(* Logix 5000 Program export KEP; software revision 30.00; part 14 of 15 *)
(* tags used below, declared in another part *)
   B256_CtoE : B256_CtoE;
   B256_CtoS : B256_CtoS;
   B256_DINTtoE : B256_DINTtoE;
   B256_EtoC : B256_EtoC;
   B256_EtoDINT : B256_EtoDINT;
   B256_EtoL : B256_EtoL;
   B256_StoC : B256_StoC;
   B256_StoC_LE : B256_StoC_LE;
   EdDSA_INTERNAL : EdDSA_INTERNAL[5];
   EdDSA_STATES : EdDSA_STATECTRL[15];
   InternalFlags : InternalFlags[5];
   InternalFlag_CreateNewKsPrime : BOOL;
   InternalFlag_KsEqualKsPrimeStatus : BOOL;
   InternalFlag_KsExists : BOOL;
   MyNodeNumber : DINT;
   POINT_DEC : POINT_DEC;
   POINT_ENC : POINT_ENC;
   POINT_MUL : POINT_MUL;
   PRN : STRING;
   PRNG : PRNG;
   PRNG_Constant : STRING;
   PRNG_Counter : LINT;
   PRNG_Seed : LINT[13];
   SHA512_SEQ : SHA512_SEQ;
   SignedMsgDest : INT;   // 0=None 1=Server 2=Client 3=All
   Temp_Processor_C1 : DINT[22];
   Temp_Processor_C10 : DINT[22];
   Temp_Processor_C11 : DINT[22];
   Temp_Processor_C12 : DINT[22];
   Temp_Processor_C2 : DINT[22];
   Temp_Processor_C3 : DINT[22];
   Temp_Processor_C4 : DINT[22];
   Temp_Processor_C5 : DINT[22];
   Temp_Processor_C6 : DINT[22];
   Temp_Processor_C7 : DINT[22];
   Temp_Processor_C8 : DINT[22];
   Temp_Processor_C9 : DINT[22];
   Temp_Processor_D1 : DINT[43];
   Temp_Processor_DINT1 : DINT[8];
   Temp_Processor_DINT2 : DINT[8];
   Temp_Processor_E1 : DINT[32];
   Temp_Processor_E2 : DINT[32];
   Temp_Processor_HASH : LINT[8];
   Temp_Processor_L : LINT[4];
   Temp_Processor_MSG : LINT[1600];
   Temp_Processor_P1 : POINT;
   Temp_Processor_P2 : POINT;
   Temp_Processor_P3 : POINT;
   Temp_Processor_P4 : POINT;
   T_INT1 : INT;
   WorkingNode : DINT;
   EdDSA_KS : DINT[8];
   EdDSA_KS_Prime : DINT[8];
   InternalFlag_KsID : LINT;
   InternalFlag_KsPrimeID : LINT;
   Wrk_InpA : DINT[2];
(* KEP, continued *)

ROUTINE PROCESSOR_STATE6   (* ladder *)
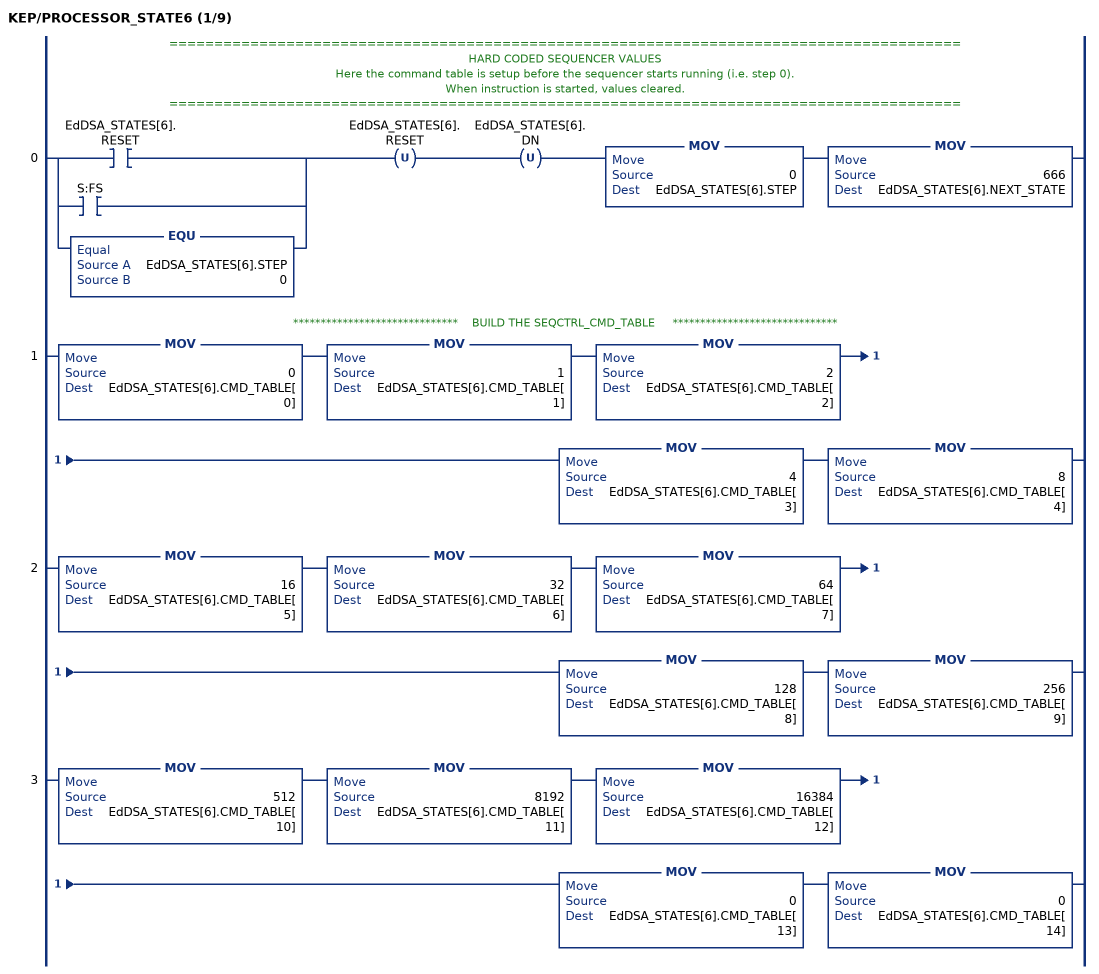
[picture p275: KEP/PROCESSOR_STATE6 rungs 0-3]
   // ========================================================================================
   // HARD CODED SEQUENCER VALUES
   // Here the command table is setup before the sequencer starts running (i.e. step 0).
   // When instruction is started, values cleared.
   // ========================================================================================
   0: [[XIC(EdDSA_STATES[6].RESET) ,XIC(S:FS) ] ,EQU(EdDSA_STATES[6].STEP,0) ]OTU(EdDSA_STATES[6].RESET)OTU(EdDSA_STATES[6].DN)MOV(0,EdDSA_STATES[6].STEP)MOV(666,EdDSA_STATES[6].NEXT_STATE);
   // ******************************    BUILD THE SEQCTRL_CMD_TABLE     ******************************
   1: MOV(0,EdDSA_STATES[6].CMD_TABLE[0])MOV(1,EdDSA_STATES[6].CMD_TABLE[1])MOV(2,EdDSA_STATES[6].CMD_TABLE[2])MOV(4,EdDSA_STATES[6].CMD_TABLE[3])MOV(8,EdDSA_STATES[6].CMD_TABLE[4]);
   2: MOV(16,EdDSA_STATES[6].CMD_TABLE[5])MOV(32,EdDSA_STATES[6].CMD_TABLE[6])MOV(64,EdDSA_STATES[6].CMD_TABLE[7])MOV(128,EdDSA_STATES[6].CMD_TABLE[8])MOV(256,EdDSA_STATES[6].CMD_TABLE[9]);
   3: MOV(512,EdDSA_STATES[6].CMD_TABLE[10])MOV(8192,EdDSA_STATES[6].CMD_TABLE[11])MOV(16384,EdDSA_STATES[6].CMD_TABLE[12])MOV(0,EdDSA_STATES[6].CMD_TABLE[13])MOV(0,EdDSA_STATES[6].CMD_TABLE[14]);
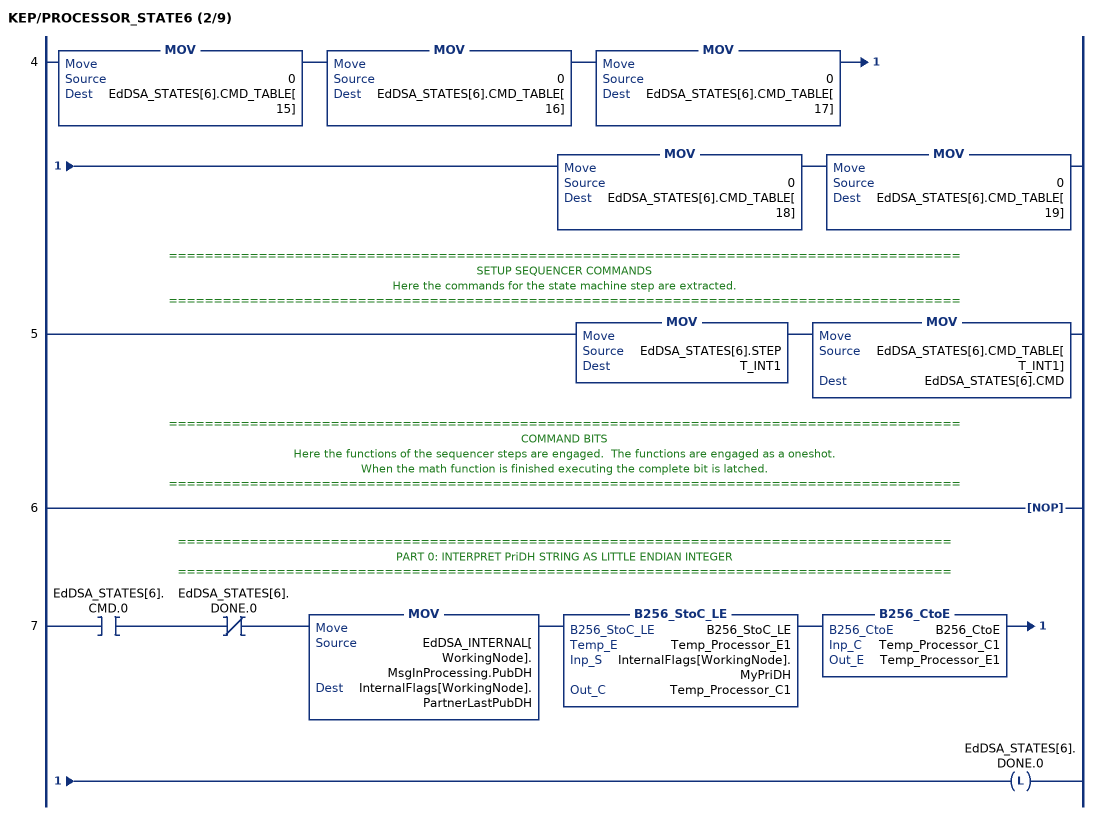
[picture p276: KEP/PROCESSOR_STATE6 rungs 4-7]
   4: MOV(0,EdDSA_STATES[6].CMD_TABLE[15])MOV(0,EdDSA_STATES[6].CMD_TABLE[16])MOV(0,EdDSA_STATES[6].CMD_TABLE[17])MOV(0,EdDSA_STATES[6].CMD_TABLE[18])MOV(0,EdDSA_STATES[6].CMD_TABLE[19]);
   // ========================================================================================
   // SETUP SEQUENCER COMMANDS
   // Here the commands for the state machine step are extracted.
   // ========================================================================================
   5: MOV(EdDSA_STATES[6].STEP,T_INT1)MOV(EdDSA_STATES[6].CMD_TABLE[T_INT1],EdDSA_STATES[6].CMD);
   // ========================================================================================
   // COMMAND BITS
   // Here the functions of the sequencer steps are engaged.  The functions are engaged as a oneshot.
   // When the math function is finished executing the complete bit is latched.
   // ========================================================================================
   6: NOP();
   // ======================================================================================
   // PART 0: INTERPRET PriDH STRING AS LITTLE ENDIAN INTEGER
   // ======================================================================================
   7: XIC(EdDSA_STATES[6].CMD.0)XIO(EdDSA_STATES[6].DONE.0)MOV(EdDSA_INTERNAL[WorkingNode].MsgInProcessing.PubDH,InternalFlags[WorkingNode].PartnerLastPubDH)B256_StoC_LE(B256_StoC_LE,Temp_Processor_E1,InternalFlags[WorkingNode].MyPriDH,Temp_Processor_C1)B256_CtoE(B256_CtoE,Temp_Processor_C1,Temp_Processor_E1)OTL(EdDSA_STATES[6].DONE.0);
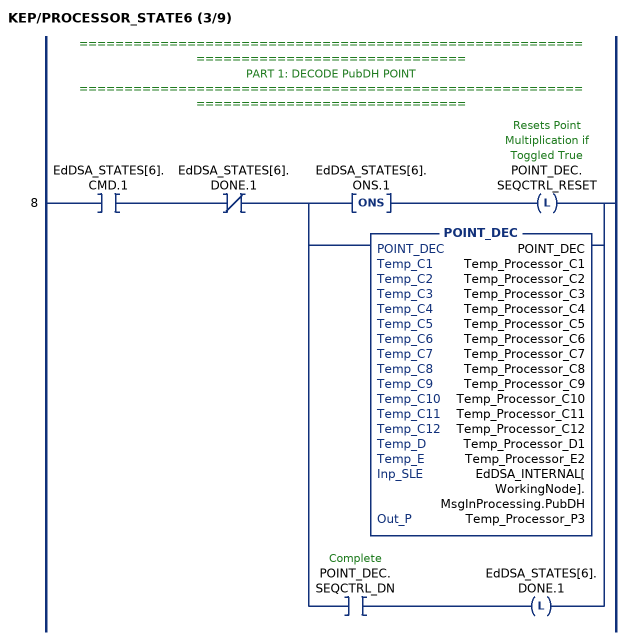
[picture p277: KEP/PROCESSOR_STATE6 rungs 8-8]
   // ======================================================================================
   // PART 1: DECODE PubDH POINT
   // ======================================================================================
   8: XIC(EdDSA_STATES[6].CMD.1)XIO(EdDSA_STATES[6].DONE.1)[ONS(EdDSA_STATES[6].ONS.1) OTL(POINT_DEC.SEQCTRL_RESET) ,POINT_DEC(POINT_DEC,Temp_Processor_C1,Temp_Processor_C2,Temp_Processor_C3,Temp_Processor_C4,Temp_Processor_C5,Temp_Processor_C6,Temp_Processor_C7,Temp_Processor_C8,Temp_Processor_C9,Temp_Processor_C10,Temp_Processor_C11,Temp_Processor_C12,Temp_Processor_D1,Temp_Processor_E2,EdDSA_INTERNAL[WorkingNode].MsgInProcessing.PubDH,Temp_Processor_P3) ,XIC(POINT_DEC.SEQCTRL_DN) OTL(EdDSA_STATES[6].DONE.1) ];
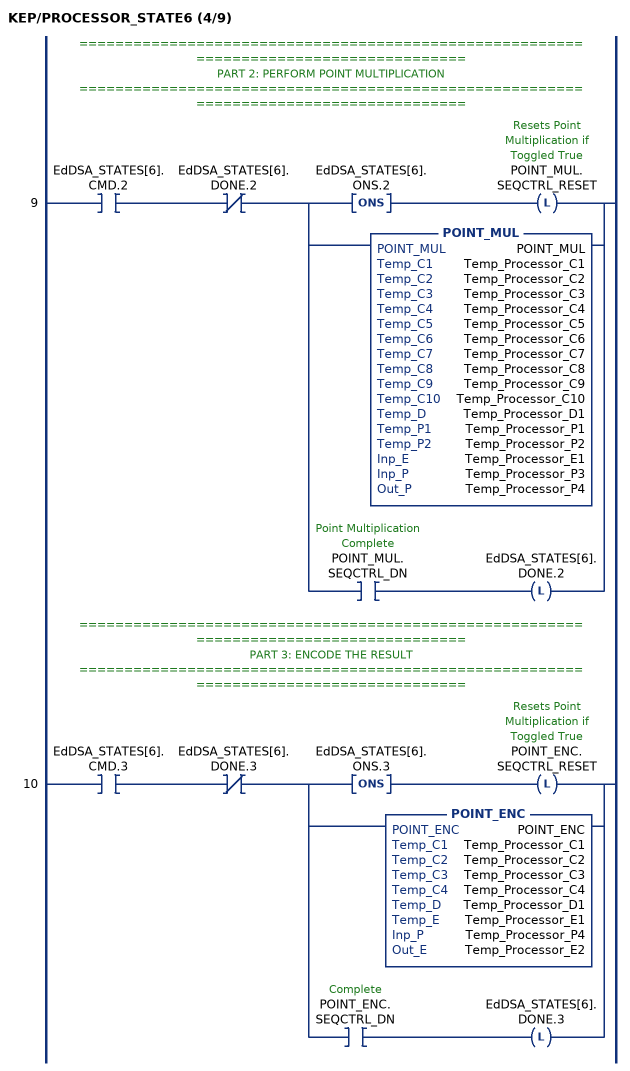
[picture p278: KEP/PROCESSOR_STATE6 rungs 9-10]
   // ======================================================================================
   // PART 2: PERFORM POINT MULTIPLICATION
   // ======================================================================================
   9: XIC(EdDSA_STATES[6].CMD.2)XIO(EdDSA_STATES[6].DONE.2)[ONS(EdDSA_STATES[6].ONS.2) OTL(POINT_MUL.SEQCTRL_RESET) ,POINT_MUL(POINT_MUL,Temp_Processor_C1,Temp_Processor_C2,Temp_Processor_C3,Temp_Processor_C4,Temp_Processor_C5,Temp_Processor_C6,Temp_Processor_C7,Temp_Processor_C8,Temp_Processor_C9,Temp_Processor_C10,Temp_Processor_D1,Temp_Processor_P1,Temp_Processor_P2,Temp_Processor_E1,Temp_Processor_P3,Temp_Processor_P4) ,XIC(POINT_MUL.SEQCTRL_DN) OTL(EdDSA_STATES[6].DONE.2) ];
   // ======================================================================================
   // PART 3: ENCODE THE RESULT
   // ======================================================================================
   10: XIC(EdDSA_STATES[6].CMD.3)XIO(EdDSA_STATES[6].DONE.3)[ONS(EdDSA_STATES[6].ONS.3) OTL(POINT_ENC.SEQCTRL_RESET) ,POINT_ENC(POINT_ENC,Temp_Processor_C1,Temp_Processor_C2,Temp_Processor_C3,Temp_Processor_C4,Temp_Processor_D1,Temp_Processor_E1,Temp_Processor_P4,Temp_Processor_E2) ,XIC(POINT_ENC.SEQCTRL_DN) OTL(EdDSA_STATES[6].DONE.3) ];
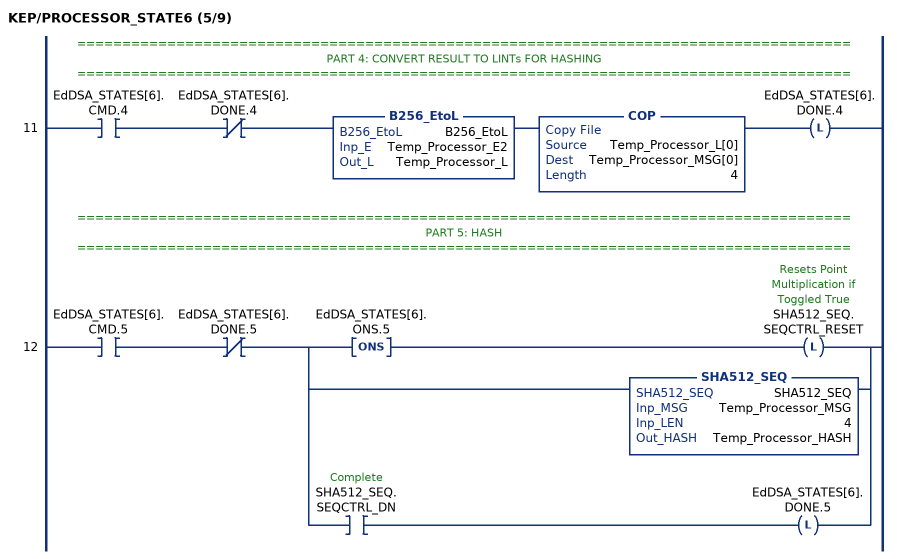
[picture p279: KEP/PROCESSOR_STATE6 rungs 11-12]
   // ======================================================================================
   // PART 4: CONVERT RESULT TO LINTs FOR HASHING
   // ======================================================================================
   11: XIC(EdDSA_STATES[6].CMD.4)XIO(EdDSA_STATES[6].DONE.4)B256_EtoL(B256_EtoL,Temp_Processor_E2,Temp_Processor_L)COP(Temp_Processor_L[0],Temp_Processor_MSG[0],4)OTL(EdDSA_STATES[6].DONE.4);
   // ======================================================================================
   // PART 5: HASH
   // ======================================================================================
   12: XIC(EdDSA_STATES[6].CMD.5)XIO(EdDSA_STATES[6].DONE.5)[ONS(EdDSA_STATES[6].ONS.5) OTL(SHA512_SEQ.SEQCTRL_RESET) ,SHA512_SEQ(SHA512_SEQ,Temp_Processor_MSG,4,Temp_Processor_HASH) ,XIC(SHA512_SEQ.SEQCTRL_DN) OTL(EdDSA_STATES[6].DONE.5) ];
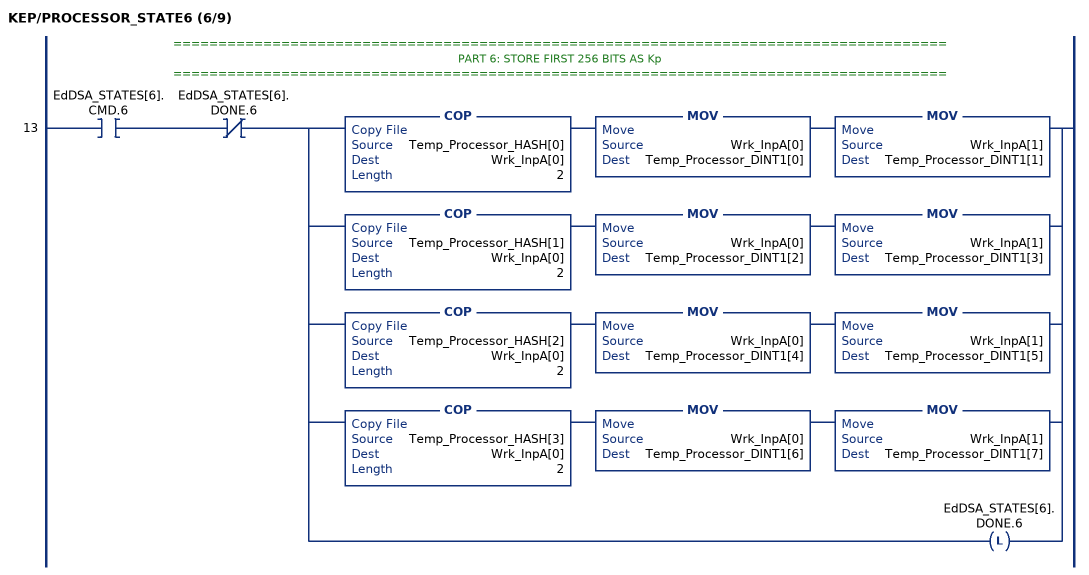
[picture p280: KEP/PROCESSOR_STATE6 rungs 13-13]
   // ======================================================================================
   // PART 6: STORE FIRST 256 BITS AS Kp
   // ======================================================================================
   13: XIC(EdDSA_STATES[6].CMD.6)XIO(EdDSA_STATES[6].DONE.6)[COP(Temp_Processor_HASH[0],Wrk_InpA[0],2) MOV(Wrk_InpA[0],Temp_Processor_DINT1[0]) MOV(Wrk_InpA[1],Temp_Processor_DINT1[1]) ,COP(Temp_Processor_HASH[1],Wrk_InpA[0],2) MOV(Wrk_InpA[0],Temp_Processor_DINT1[2]) MOV(Wrk_InpA[1],Temp_Processor_DINT1[3]) ,COP(Temp_Processor_HASH[2],Wrk_InpA[0],2) MOV(Wrk_InpA[0],Temp_Processor_DINT1[4]) MOV(Wrk_InpA[1],Temp_Processor_DINT1[5]) ,COP(Temp_Processor_HASH[3],Wrk_InpA[0],2) MOV(Wrk_InpA[0],Temp_Processor_DINT1[6]) MOV(Wrk_InpA[1],Temp_Processor_DINT1[7]) ,OTL(EdDSA_STATES[6].DONE.6) ];
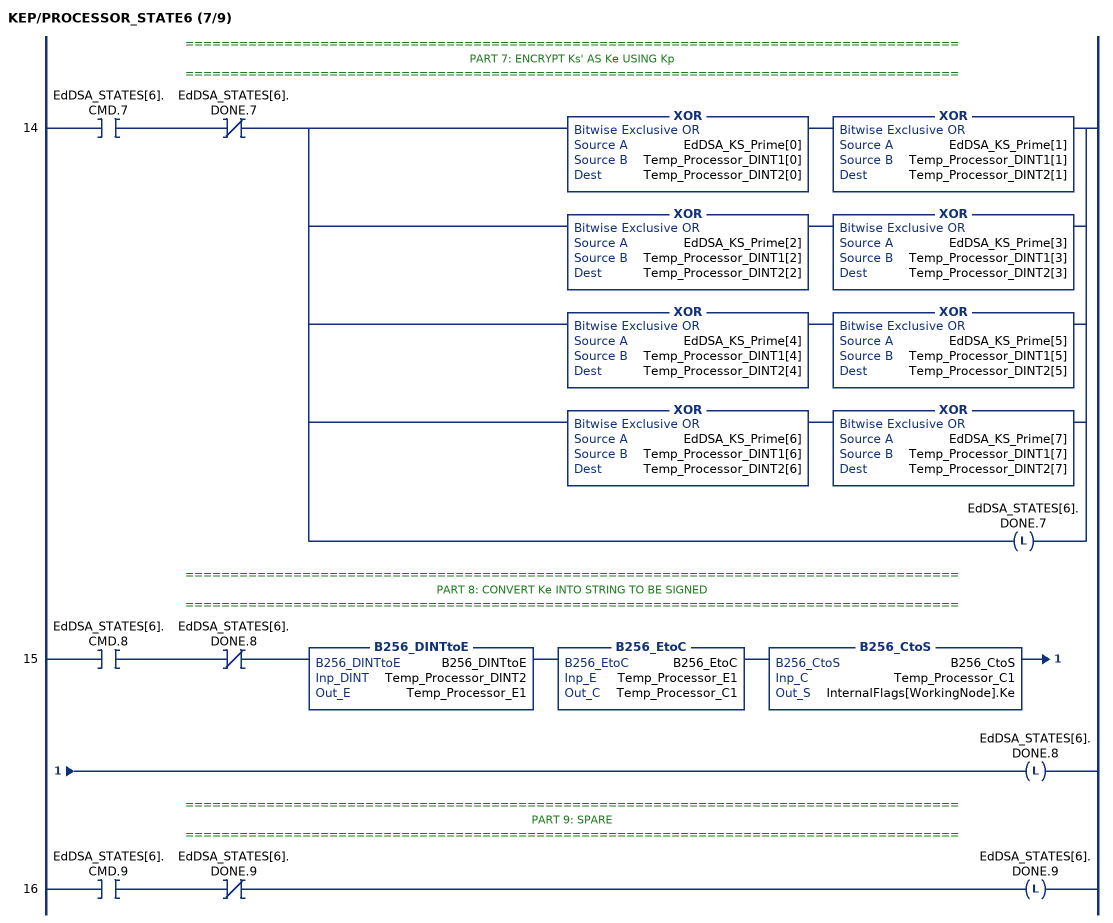
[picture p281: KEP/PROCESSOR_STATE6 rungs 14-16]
   // ======================================================================================
   // PART 7: ENCRYPT Ks' AS Ke USING Kp
   // ======================================================================================
   14: XIC(EdDSA_STATES[6].CMD.7)XIO(EdDSA_STATES[6].DONE.7)[XOR(EdDSA_KS_Prime[0],Temp_Processor_DINT1[0],Temp_Processor_DINT2[0]) XOR(EdDSA_KS_Prime[1],Temp_Processor_DINT1[1],Temp_Processor_DINT2[1]) ,XOR(EdDSA_KS_Prime[2],Temp_Processor_DINT1[2],Temp_Processor_DINT2[2]) XOR(EdDSA_KS_Prime[3],Temp_Processor_DINT1[3],Temp_Processor_DINT2[3]) ,XOR(EdDSA_KS_Prime[4],Temp_Processor_DINT1[4],Temp_Processor_DINT2[4]) XOR(EdDSA_KS_Prime[5],Temp_Processor_DINT1[5],Temp_Processor_DINT2[5]) ,XOR(EdDSA_KS_Prime[6],Temp_Processor_DINT1[6],Temp_Processor_DINT2[6]) XOR(EdDSA_KS_Prime[7],Temp_Processor_DINT1[7],Temp_Processor_DINT2[7]) ,OTL(EdDSA_STATES[6].DONE.7) ];
   // ======================================================================================
   // PART 8: CONVERT Ke INTO STRING TO BE SIGNED
   // ======================================================================================
   15: XIC(EdDSA_STATES[6].CMD.8)XIO(EdDSA_STATES[6].DONE.8)B256_DINTtoE(B256_DINTtoE,Temp_Processor_DINT2,Temp_Processor_E1)B256_EtoC(B256_EtoC,Temp_Processor_E1,Temp_Processor_C1)B256_CtoS(B256_CtoS,Temp_Processor_C1,InternalFlags[WorkingNode].Ke)OTL(EdDSA_STATES[6].DONE.8);
   // ======================================================================================
   // PART 9: SPARE
   // ======================================================================================
   16: XIC(EdDSA_STATES[6].CMD.9)XIO(EdDSA_STATES[6].DONE.9)OTL(EdDSA_STATES[6].DONE.9);
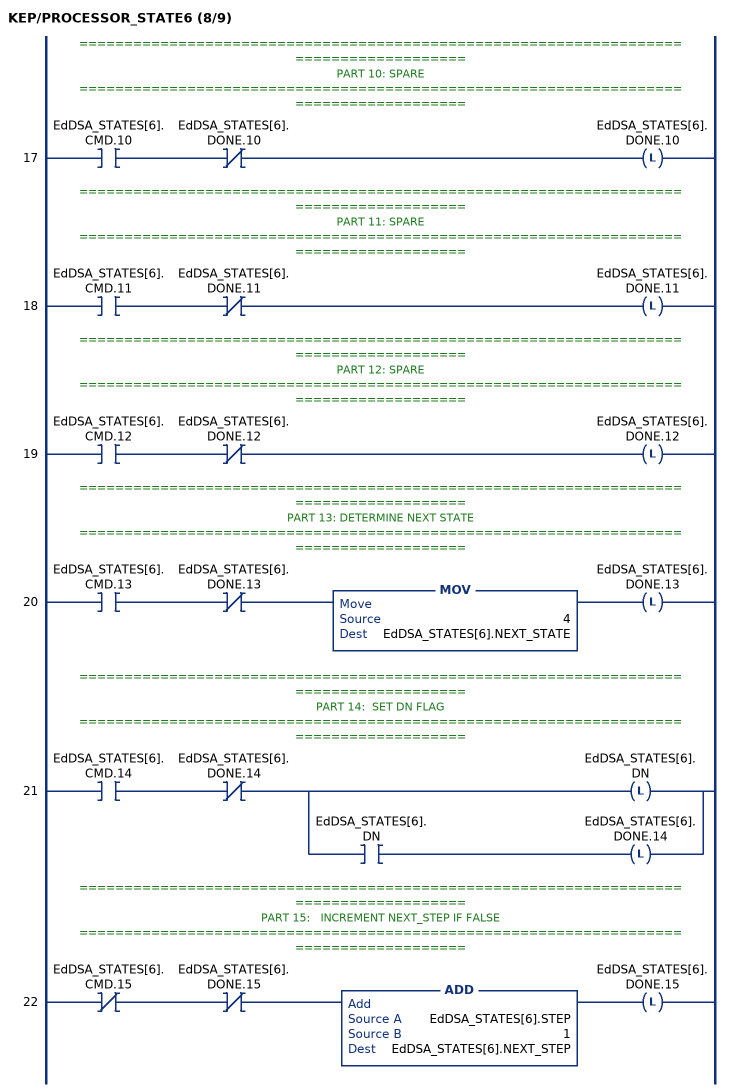
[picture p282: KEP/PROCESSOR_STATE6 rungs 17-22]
   // ======================================================================================
   // PART 10: SPARE
   // ======================================================================================
   17: XIC(EdDSA_STATES[6].CMD.10)XIO(EdDSA_STATES[6].DONE.10)OTL(EdDSA_STATES[6].DONE.10);
   // ======================================================================================
   // PART 11: SPARE
   // ======================================================================================
   18: XIC(EdDSA_STATES[6].CMD.11)XIO(EdDSA_STATES[6].DONE.11)OTL(EdDSA_STATES[6].DONE.11);
   // ======================================================================================
   // PART 12: SPARE
   // ======================================================================================
   19: XIC(EdDSA_STATES[6].CMD.12)XIO(EdDSA_STATES[6].DONE.12)OTL(EdDSA_STATES[6].DONE.12);
   // ======================================================================================
   // PART 13: DETERMINE NEXT STATE
   // ======================================================================================
   20: XIC(EdDSA_STATES[6].CMD.13)XIO(EdDSA_STATES[6].DONE.13)MOV(4,EdDSA_STATES[6].NEXT_STATE)OTL(EdDSA_STATES[6].DONE.13);
   // ======================================================================================
   // PART 14:  SET DN FLAG
   // ======================================================================================
   21: XIC(EdDSA_STATES[6].CMD.14)XIO(EdDSA_STATES[6].DONE.14)[OTL(EdDSA_STATES[6].DN) ,XIC(EdDSA_STATES[6].DN) OTL(EdDSA_STATES[6].DONE.14) ];
   // ======================================================================================
   // PART 15:   INCREMENT NEXT_STEP IF FALSE
   // ======================================================================================
   22: XIO(EdDSA_STATES[6].CMD.15)XIO(EdDSA_STATES[6].DONE.15)ADD(EdDSA_STATES[6].STEP,1,EdDSA_STATES[6].NEXT_STEP)OTL(EdDSA_STATES[6].DONE.15);
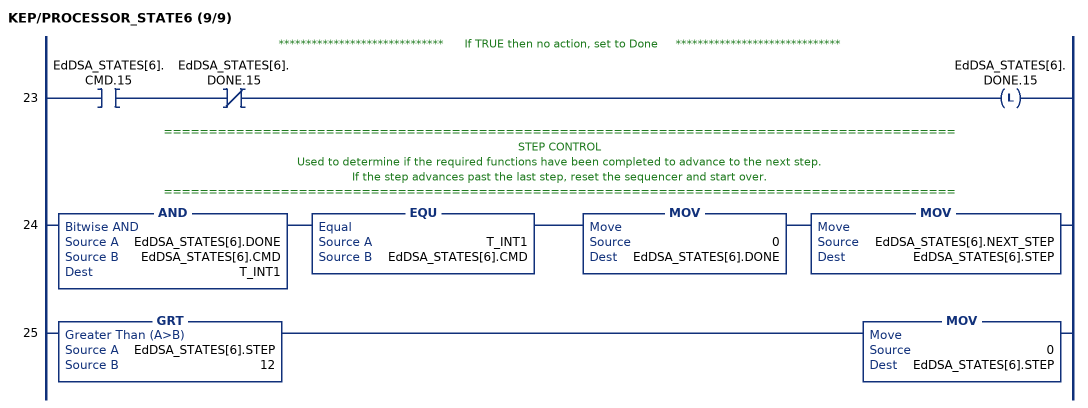
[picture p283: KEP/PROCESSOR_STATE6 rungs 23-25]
   // ******************************      If TRUE then no action, set to Done     ******************************
   23: XIC(EdDSA_STATES[6].CMD.15)XIO(EdDSA_STATES[6].DONE.15)OTL(EdDSA_STATES[6].DONE.15);
   // ========================================================================================
   // STEP CONTROL
   // Used to determine if the required functions have been completed to advance to the next step.
   // If the step advances past the last step, reset the sequencer and start over.
   // ========================================================================================
   24: AND(EdDSA_STATES[6].DONE,EdDSA_STATES[6].CMD,T_INT1)EQU(T_INT1,EdDSA_STATES[6].CMD)MOV(0,EdDSA_STATES[6].DONE)MOV(EdDSA_STATES[6].NEXT_STEP,EdDSA_STATES[6].STEP);
   25: GRT(EdDSA_STATES[6].STEP,12)MOV(0,EdDSA_STATES[6].STEP);
END_ROUTINE

ROUTINE PROCESSOR_STATE7   (* ladder *)
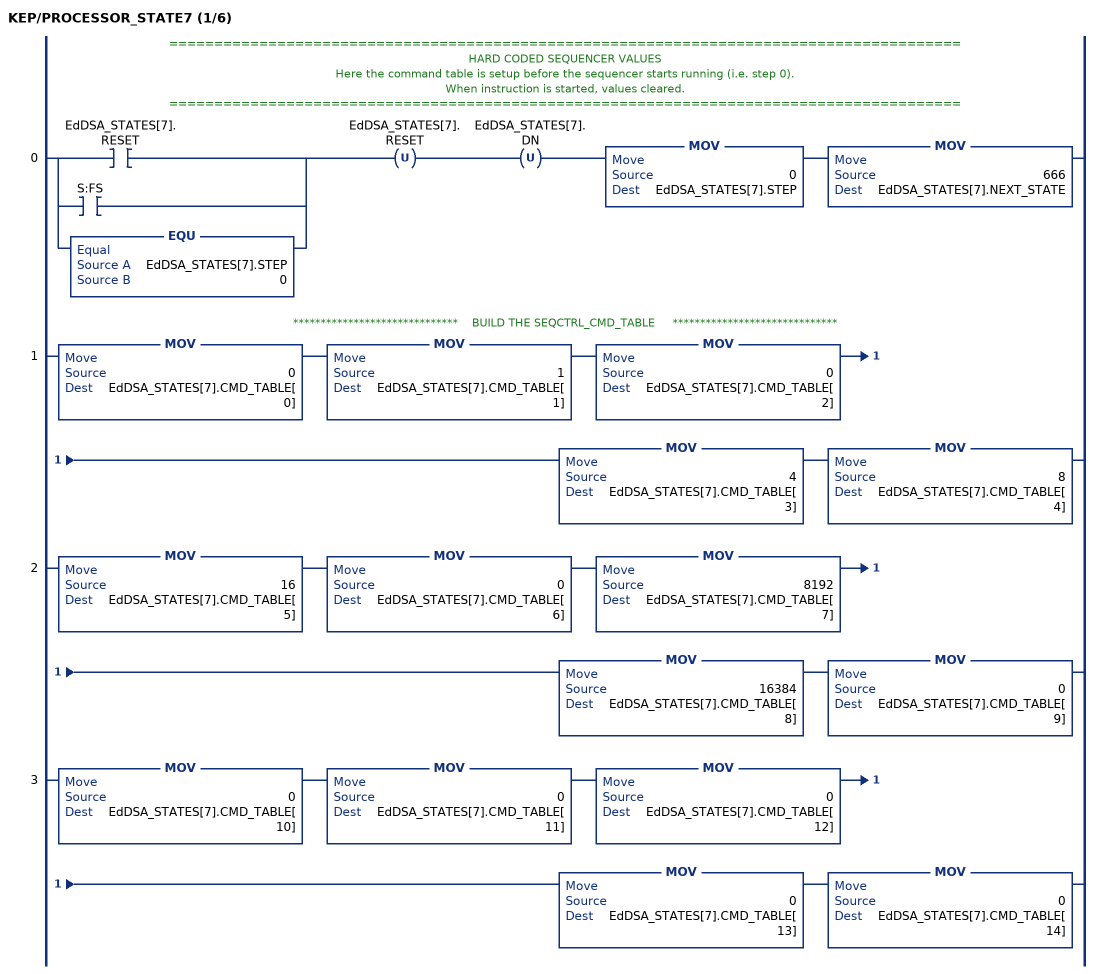
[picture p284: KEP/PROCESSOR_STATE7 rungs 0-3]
   // ========================================================================================
   // HARD CODED SEQUENCER VALUES
   // Here the command table is setup before the sequencer starts running (i.e. step 0).
   // When instruction is started, values cleared.
   // ========================================================================================
   0: [[XIC(EdDSA_STATES[7].RESET) ,XIC(S:FS) ] ,EQU(EdDSA_STATES[7].STEP,0) ]OTU(EdDSA_STATES[7].RESET)OTU(EdDSA_STATES[7].DN)MOV(0,EdDSA_STATES[7].STEP)MOV(666,EdDSA_STATES[7].NEXT_STATE);
   // ******************************    BUILD THE SEQCTRL_CMD_TABLE     ******************************
   1: MOV(0,EdDSA_STATES[7].CMD_TABLE[0])MOV(1,EdDSA_STATES[7].CMD_TABLE[1])MOV(0,EdDSA_STATES[7].CMD_TABLE[2])MOV(4,EdDSA_STATES[7].CMD_TABLE[3])MOV(8,EdDSA_STATES[7].CMD_TABLE[4]);
   2: MOV(16,EdDSA_STATES[7].CMD_TABLE[5])MOV(0,EdDSA_STATES[7].CMD_TABLE[6])MOV(8192,EdDSA_STATES[7].CMD_TABLE[7])MOV(16384,EdDSA_STATES[7].CMD_TABLE[8])MOV(0,EdDSA_STATES[7].CMD_TABLE[9]);
   3: MOV(0,EdDSA_STATES[7].CMD_TABLE[10])MOV(0,EdDSA_STATES[7].CMD_TABLE[11])MOV(0,EdDSA_STATES[7].CMD_TABLE[12])MOV(0,EdDSA_STATES[7].CMD_TABLE[13])MOV(0,EdDSA_STATES[7].CMD_TABLE[14]);
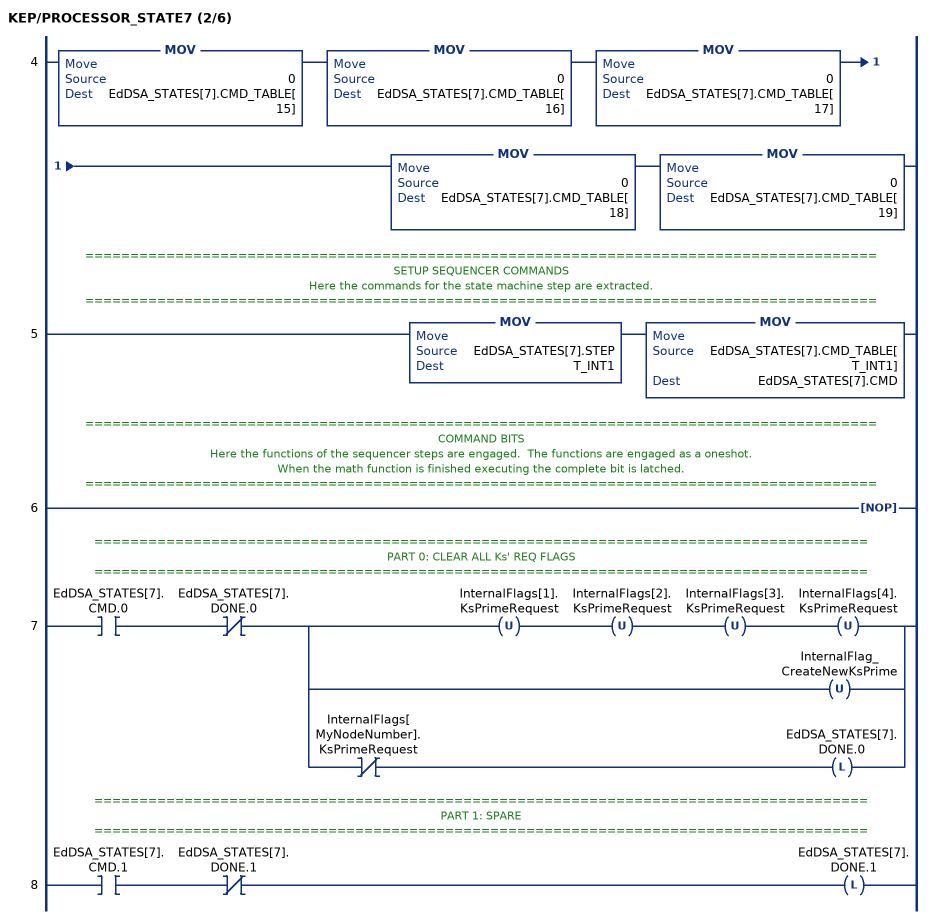
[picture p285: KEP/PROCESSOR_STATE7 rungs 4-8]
   4: MOV(0,EdDSA_STATES[7].CMD_TABLE[15])MOV(0,EdDSA_STATES[7].CMD_TABLE[16])MOV(0,EdDSA_STATES[7].CMD_TABLE[17])MOV(0,EdDSA_STATES[7].CMD_TABLE[18])MOV(0,EdDSA_STATES[7].CMD_TABLE[19]);
   // ========================================================================================
   // SETUP SEQUENCER COMMANDS
   // Here the commands for the state machine step are extracted.
   // ========================================================================================
   5: MOV(EdDSA_STATES[7].STEP,T_INT1)MOV(EdDSA_STATES[7].CMD_TABLE[T_INT1],EdDSA_STATES[7].CMD);
   // ========================================================================================
   // COMMAND BITS
   // Here the functions of the sequencer steps are engaged.  The functions are engaged as a oneshot.
   // When the math function is finished executing the complete bit is latched.
   // ========================================================================================
   6: NOP();
   // ======================================================================================
   // PART 0: CLEAR ALL Ks' REQ FLAGS
   // ======================================================================================
   7: XIC(EdDSA_STATES[7].CMD.0)XIO(EdDSA_STATES[7].DONE.0)[OTU(InternalFlags[1].KsPrimeRequest) OTU(InternalFlags[2].KsPrimeRequest) OTU(InternalFlags[3].KsPrimeRequest) OTU(InternalFlags[4].KsPrimeRequest) ,OTU(InternalFlag_CreateNewKsPrime) ,XIO(InternalFlags[MyNodeNumber].KsPrimeRequest) OTL(EdDSA_STATES[7].DONE.0) ];
   // ======================================================================================
   // PART 1: SPARE
   // ======================================================================================
   8: XIC(EdDSA_STATES[7].CMD.1)XIO(EdDSA_STATES[7].DONE.1)OTL(EdDSA_STATES[7].DONE.1);
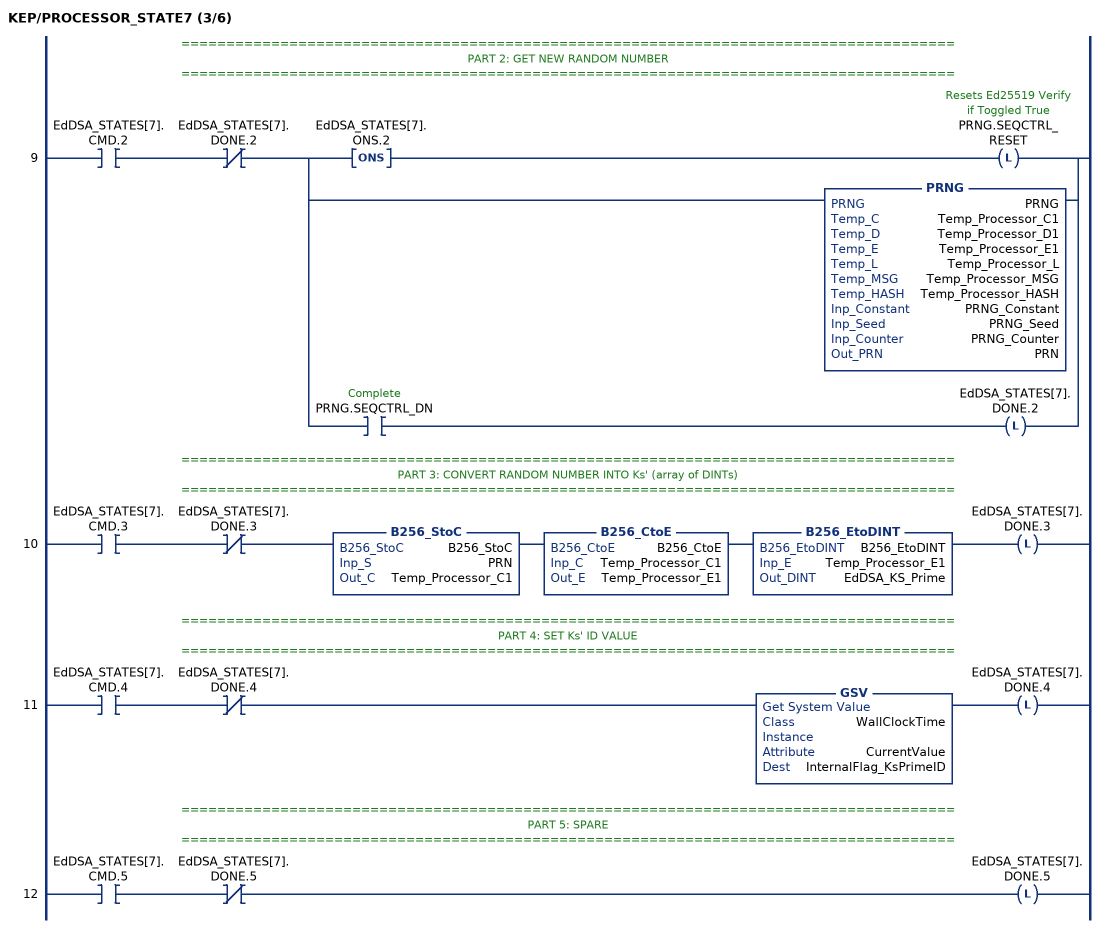
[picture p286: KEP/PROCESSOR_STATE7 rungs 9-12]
   // ======================================================================================
   // PART 2: GET NEW RANDOM NUMBER
   // ======================================================================================
   9: XIC(EdDSA_STATES[7].CMD.2)XIO(EdDSA_STATES[7].DONE.2)[ONS(EdDSA_STATES[7].ONS.2) OTL(PRNG.SEQCTRL_RESET) ,PRNG(PRNG,Temp_Processor_C1,Temp_Processor_D1,Temp_Processor_E1,Temp_Processor_L,Temp_Processor_MSG,Temp_Processor_HASH,PRNG_Constant,PRNG_Seed,PRNG_Counter,PRN) ,XIC(PRNG.SEQCTRL_DN) OTL(EdDSA_STATES[7].DONE.2) ];
   // ======================================================================================
   // PART 3: CONVERT RANDOM NUMBER INTO Ks' (array of DINTs)
   // ======================================================================================
   10: XIC(EdDSA_STATES[7].CMD.3)XIO(EdDSA_STATES[7].DONE.3)B256_StoC(B256_StoC,PRN,Temp_Processor_C1)B256_CtoE(B256_CtoE,Temp_Processor_C1,Temp_Processor_E1)B256_EtoDINT(B256_EtoDINT,Temp_Processor_E1,EdDSA_KS_Prime)OTL(EdDSA_STATES[7].DONE.3);
   // ======================================================================================
   // PART 4: SET Ks' ID VALUE
   // ======================================================================================
   11: XIC(EdDSA_STATES[7].CMD.4)XIO(EdDSA_STATES[7].DONE.4)GSV(WallClockTime,,CurrentValue,InternalFlag_KsPrimeID)OTL(EdDSA_STATES[7].DONE.4);
   // ======================================================================================
   // PART 5: SPARE
   // ======================================================================================
   12: XIC(EdDSA_STATES[7].CMD.5)XIO(EdDSA_STATES[7].DONE.5)OTL(EdDSA_STATES[7].DONE.5);
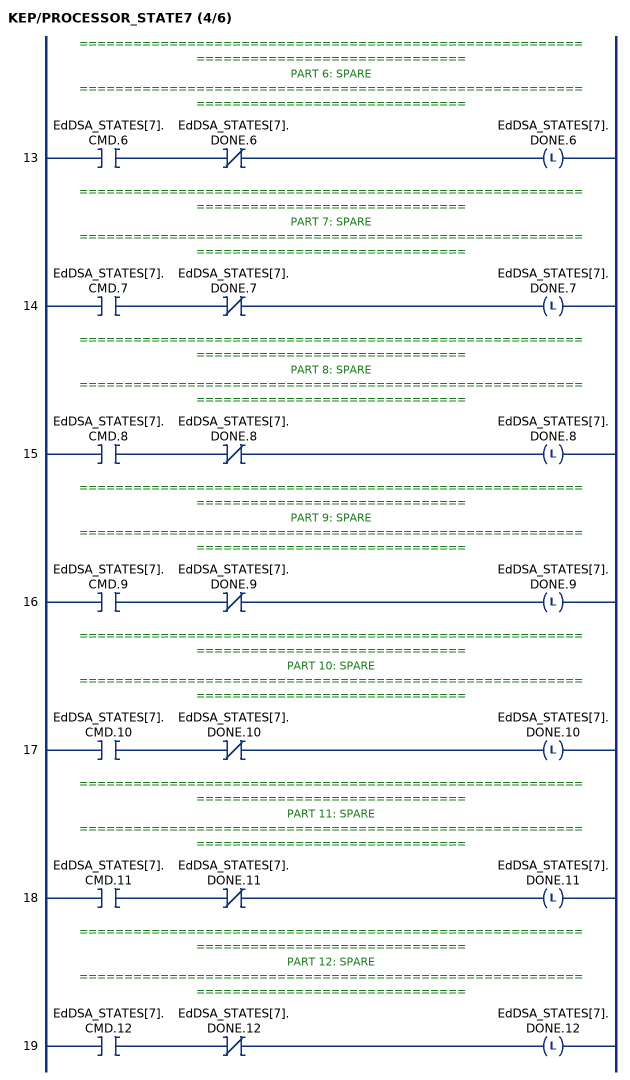
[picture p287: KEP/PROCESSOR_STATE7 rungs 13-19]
   // ======================================================================================
   // PART 6: SPARE
   // ======================================================================================
   13: XIC(EdDSA_STATES[7].CMD.6)XIO(EdDSA_STATES[7].DONE.6)OTL(EdDSA_STATES[7].DONE.6);
   // ======================================================================================
   // PART 7: SPARE
   // ======================================================================================
   14: XIC(EdDSA_STATES[7].CMD.7)XIO(EdDSA_STATES[7].DONE.7)OTL(EdDSA_STATES[7].DONE.7);
   // ======================================================================================
   // PART 8: SPARE
   // ======================================================================================
   15: XIC(EdDSA_STATES[7].CMD.8)XIO(EdDSA_STATES[7].DONE.8)OTL(EdDSA_STATES[7].DONE.8);
   // ======================================================================================
   // PART 9: SPARE
   // ======================================================================================
   16: XIC(EdDSA_STATES[7].CMD.9)XIO(EdDSA_STATES[7].DONE.9)OTL(EdDSA_STATES[7].DONE.9);
   // ======================================================================================
   // PART 10: SPARE
   // ======================================================================================
   17: XIC(EdDSA_STATES[7].CMD.10)XIO(EdDSA_STATES[7].DONE.10)OTL(EdDSA_STATES[7].DONE.10);
   // ======================================================================================
   // PART 11: SPARE
   // ======================================================================================
   18: XIC(EdDSA_STATES[7].CMD.11)XIO(EdDSA_STATES[7].DONE.11)OTL(EdDSA_STATES[7].DONE.11);
   // ======================================================================================
   // PART 12: SPARE
   // ======================================================================================
   19: XIC(EdDSA_STATES[7].CMD.12)XIO(EdDSA_STATES[7].DONE.12)OTL(EdDSA_STATES[7].DONE.12);
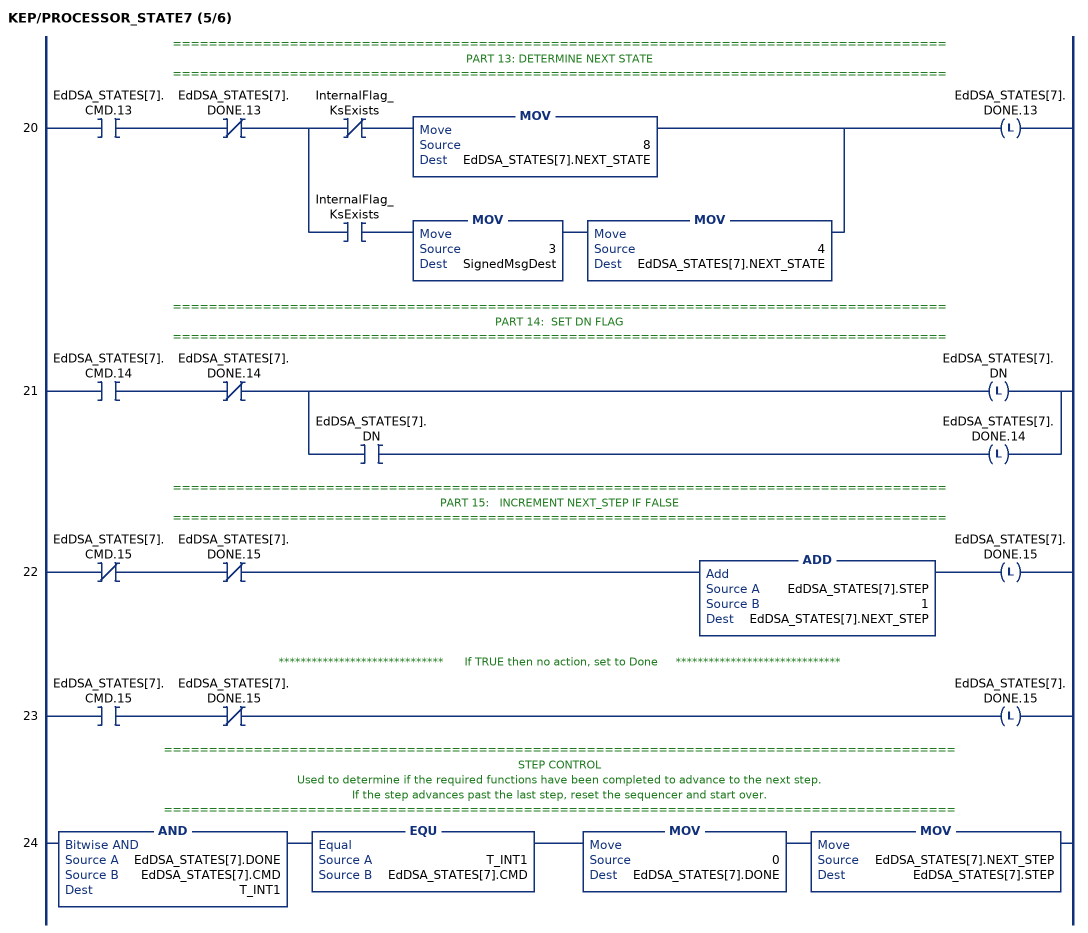
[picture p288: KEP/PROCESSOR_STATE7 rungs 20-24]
   // ======================================================================================
   // PART 13: DETERMINE NEXT STATE
   // ======================================================================================
   20: XIC(EdDSA_STATES[7].CMD.13)XIO(EdDSA_STATES[7].DONE.13)[XIO(InternalFlag_KsExists) MOV(8,EdDSA_STATES[7].NEXT_STATE) ,XIC(InternalFlag_KsExists) MOV(3,SignedMsgDest) MOV(4,EdDSA_STATES[7].NEXT_STATE) ]OTL(EdDSA_STATES[7].DONE.13);
   // ======================================================================================
   // PART 14:  SET DN FLAG
   // ======================================================================================
   21: XIC(EdDSA_STATES[7].CMD.14)XIO(EdDSA_STATES[7].DONE.14)[OTL(EdDSA_STATES[7].DN) ,XIC(EdDSA_STATES[7].DN) OTL(EdDSA_STATES[7].DONE.14) ];
   // ======================================================================================
   // PART 15:   INCREMENT NEXT_STEP IF FALSE
   // ======================================================================================
   22: XIO(EdDSA_STATES[7].CMD.15)XIO(EdDSA_STATES[7].DONE.15)ADD(EdDSA_STATES[7].STEP,1,EdDSA_STATES[7].NEXT_STEP)OTL(EdDSA_STATES[7].DONE.15);
   // ******************************      If TRUE then no action, set to Done     ******************************
   23: XIC(EdDSA_STATES[7].CMD.15)XIO(EdDSA_STATES[7].DONE.15)OTL(EdDSA_STATES[7].DONE.15);
   // ========================================================================================
   // STEP CONTROL
   // Used to determine if the required functions have been completed to advance to the next step.
   // If the step advances past the last step, reset the sequencer and start over.
   // ========================================================================================
   24: AND(EdDSA_STATES[7].DONE,EdDSA_STATES[7].CMD,T_INT1)EQU(T_INT1,EdDSA_STATES[7].CMD)MOV(0,EdDSA_STATES[7].DONE)MOV(EdDSA_STATES[7].NEXT_STEP,EdDSA_STATES[7].STEP);
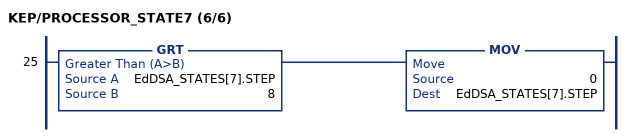
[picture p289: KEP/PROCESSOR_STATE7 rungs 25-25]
   25: GRT(EdDSA_STATES[7].STEP,8)MOV(0,EdDSA_STATES[7].STEP);
END_ROUTINE

ROUTINE PROCESSOR_STATE8   (* ladder *)
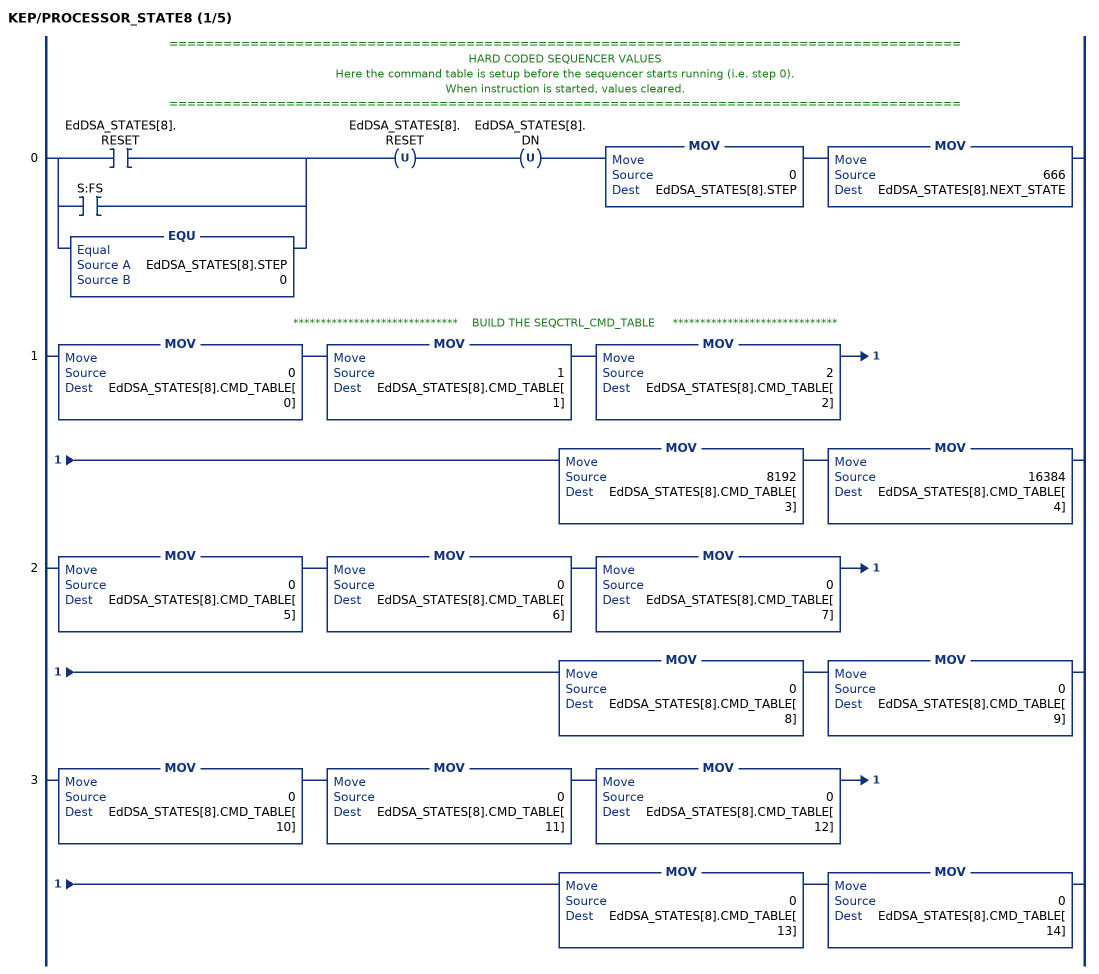
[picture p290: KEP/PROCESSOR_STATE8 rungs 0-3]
   // ========================================================================================
   // HARD CODED SEQUENCER VALUES
   // Here the command table is setup before the sequencer starts running (i.e. step 0).
   // When instruction is started, values cleared.
   // ========================================================================================
   0: [[XIC(EdDSA_STATES[8].RESET) ,XIC(S:FS) ] ,EQU(EdDSA_STATES[8].STEP,0) ]OTU(EdDSA_STATES[8].RESET)OTU(EdDSA_STATES[8].DN)MOV(0,EdDSA_STATES[8].STEP)MOV(666,EdDSA_STATES[8].NEXT_STATE);
   // ******************************    BUILD THE SEQCTRL_CMD_TABLE     ******************************
   1: MOV(0,EdDSA_STATES[8].CMD_TABLE[0])MOV(1,EdDSA_STATES[8].CMD_TABLE[1])MOV(2,EdDSA_STATES[8].CMD_TABLE[2])MOV(8192,EdDSA_STATES[8].CMD_TABLE[3])MOV(16384,EdDSA_STATES[8].CMD_TABLE[4]);
   2: MOV(0,EdDSA_STATES[8].CMD_TABLE[5])MOV(0,EdDSA_STATES[8].CMD_TABLE[6])MOV(0,EdDSA_STATES[8].CMD_TABLE[7])MOV(0,EdDSA_STATES[8].CMD_TABLE[8])MOV(0,EdDSA_STATES[8].CMD_TABLE[9]);
   3: MOV(0,EdDSA_STATES[8].CMD_TABLE[10])MOV(0,EdDSA_STATES[8].CMD_TABLE[11])MOV(0,EdDSA_STATES[8].CMD_TABLE[12])MOV(0,EdDSA_STATES[8].CMD_TABLE[13])MOV(0,EdDSA_STATES[8].CMD_TABLE[14]);
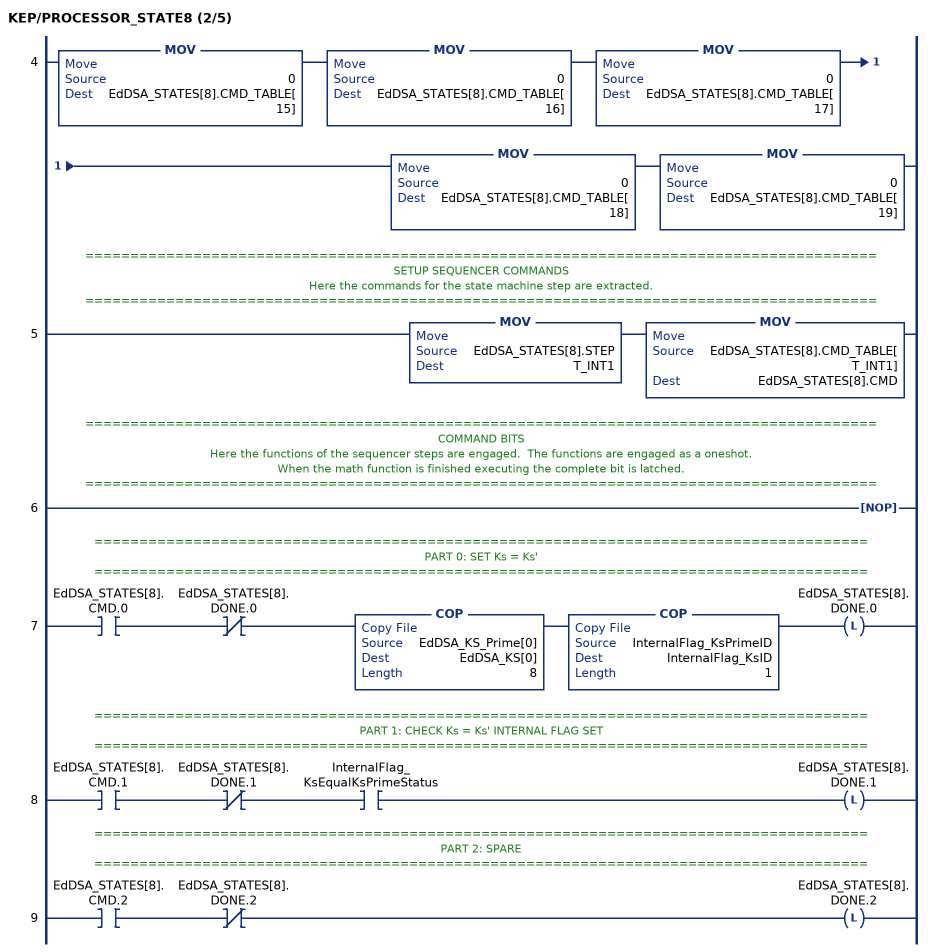
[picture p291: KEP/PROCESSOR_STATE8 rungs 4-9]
   4: MOV(0,EdDSA_STATES[8].CMD_TABLE[15])MOV(0,EdDSA_STATES[8].CMD_TABLE[16])MOV(0,EdDSA_STATES[8].CMD_TABLE[17])MOV(0,EdDSA_STATES[8].CMD_TABLE[18])MOV(0,EdDSA_STATES[8].CMD_TABLE[19]);
   // ========================================================================================
   // SETUP SEQUENCER COMMANDS
   // Here the commands for the state machine step are extracted.
   // ========================================================================================
   5: MOV(EdDSA_STATES[8].STEP,T_INT1)MOV(EdDSA_STATES[8].CMD_TABLE[T_INT1],EdDSA_STATES[8].CMD);
   // ========================================================================================
   // COMMAND BITS
   // Here the functions of the sequencer steps are engaged.  The functions are engaged as a oneshot.
   // When the math function is finished executing the complete bit is latched.
   // ========================================================================================
   6: NOP();
   // ======================================================================================
   // PART 0: SET Ks = Ks'
   // ======================================================================================
   7: XIC(EdDSA_STATES[8].CMD.0)XIO(EdDSA_STATES[8].DONE.0)COP(EdDSA_KS_Prime[0],EdDSA_KS[0],8)COP(InternalFlag_KsPrimeID,InternalFlag_KsID,1)OTL(EdDSA_STATES[8].DONE.0);
   // ======================================================================================
   // PART 1: CHECK Ks = Ks' INTERNAL FLAG SET
   // ======================================================================================
   8: XIC(EdDSA_STATES[8].CMD.1)XIO(EdDSA_STATES[8].DONE.1)XIC(InternalFlag_KsEqualKsPrimeStatus)OTL(EdDSA_STATES[8].DONE.1);
   // ======================================================================================
   // PART 2: SPARE
   // ======================================================================================
   9: XIC(EdDSA_STATES[8].CMD.2)XIO(EdDSA_STATES[8].DONE.2)OTL(EdDSA_STATES[8].DONE.2);
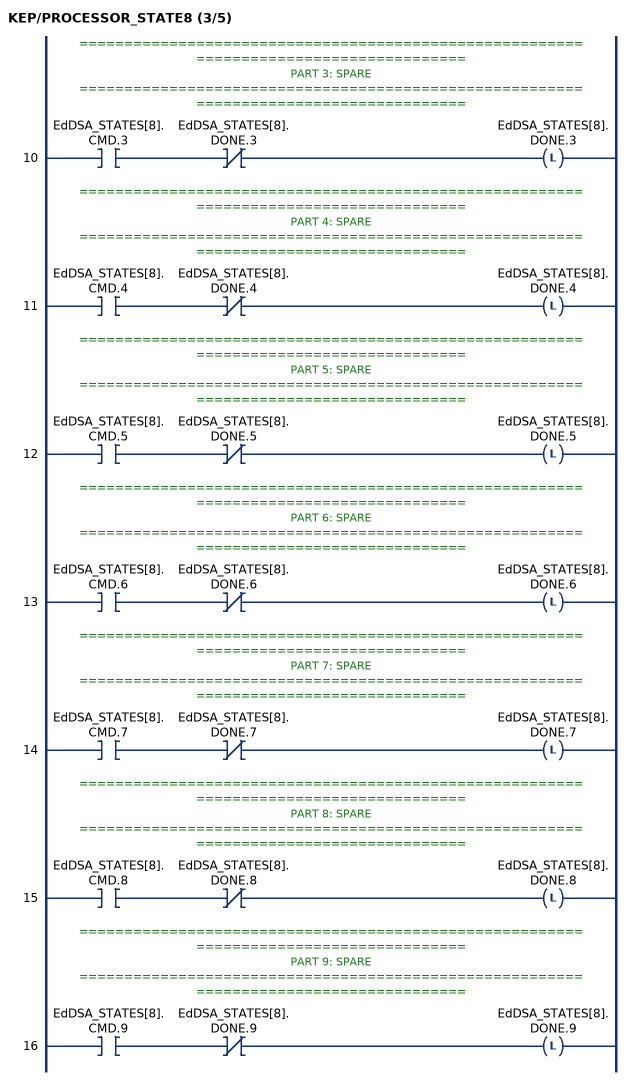
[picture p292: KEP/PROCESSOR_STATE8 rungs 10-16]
   // ======================================================================================
   // PART 3: SPARE
   // ======================================================================================
   10: XIC(EdDSA_STATES[8].CMD.3)XIO(EdDSA_STATES[8].DONE.3)OTL(EdDSA_STATES[8].DONE.3);
   // ======================================================================================
   // PART 4: SPARE
   // ======================================================================================
   11: XIC(EdDSA_STATES[8].CMD.4)XIO(EdDSA_STATES[8].DONE.4)OTL(EdDSA_STATES[8].DONE.4);
   // ======================================================================================
   // PART 5: SPARE
   // ======================================================================================
   12: XIC(EdDSA_STATES[8].CMD.5)XIO(EdDSA_STATES[8].DONE.5)OTL(EdDSA_STATES[8].DONE.5);
   // ======================================================================================
   // PART 6: SPARE
   // ======================================================================================
   13: XIC(EdDSA_STATES[8].CMD.6)XIO(EdDSA_STATES[8].DONE.6)OTL(EdDSA_STATES[8].DONE.6);
   // ======================================================================================
   // PART 7: SPARE
   // ======================================================================================
   14: XIC(EdDSA_STATES[8].CMD.7)XIO(EdDSA_STATES[8].DONE.7)OTL(EdDSA_STATES[8].DONE.7);
   // ======================================================================================
   // PART 8: SPARE
   // ======================================================================================
   15: XIC(EdDSA_STATES[8].CMD.8)XIO(EdDSA_STATES[8].DONE.8)OTL(EdDSA_STATES[8].DONE.8);
   // ======================================================================================
   // PART 9: SPARE
   // ======================================================================================
   16: XIC(EdDSA_STATES[8].CMD.9)XIO(EdDSA_STATES[8].DONE.9)OTL(EdDSA_STATES[8].DONE.9);
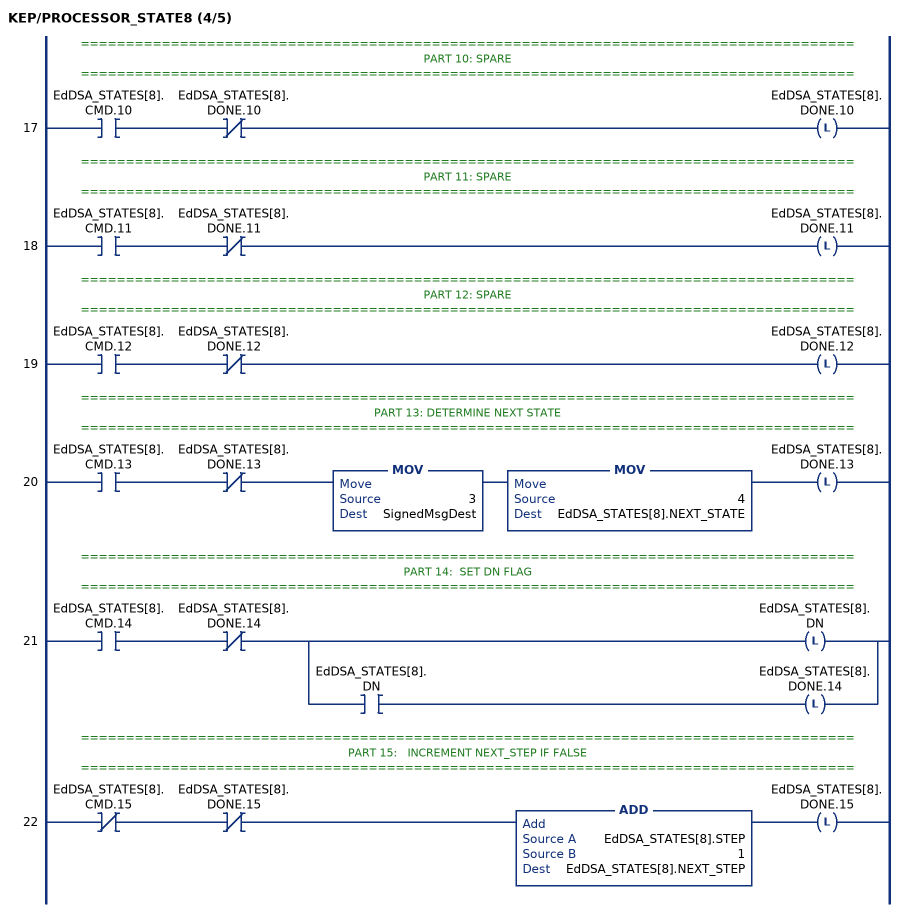
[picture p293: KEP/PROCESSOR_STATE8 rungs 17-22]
   // ======================================================================================
   // PART 10: SPARE
   // ======================================================================================
   17: XIC(EdDSA_STATES[8].CMD.10)XIO(EdDSA_STATES[8].DONE.10)OTL(EdDSA_STATES[8].DONE.10);
   // ======================================================================================
   // PART 11: SPARE
   // ======================================================================================
   18: XIC(EdDSA_STATES[8].CMD.11)XIO(EdDSA_STATES[8].DONE.11)OTL(EdDSA_STATES[8].DONE.11);
   // ======================================================================================
   // PART 12: SPARE
   // ======================================================================================
   19: XIC(EdDSA_STATES[8].CMD.12)XIO(EdDSA_STATES[8].DONE.12)OTL(EdDSA_STATES[8].DONE.12);
   // ======================================================================================
   // PART 13: DETERMINE NEXT STATE
   // ======================================================================================
   20: XIC(EdDSA_STATES[8].CMD.13)XIO(EdDSA_STATES[8].DONE.13)MOV(3,SignedMsgDest)MOV(4,EdDSA_STATES[8].NEXT_STATE)OTL(EdDSA_STATES[8].DONE.13);
   // ======================================================================================
   // PART 14:  SET DN FLAG
   // ======================================================================================
   21: XIC(EdDSA_STATES[8].CMD.14)XIO(EdDSA_STATES[8].DONE.14)[OTL(EdDSA_STATES[8].DN) ,XIC(EdDSA_STATES[8].DN) OTL(EdDSA_STATES[8].DONE.14) ];
   // ======================================================================================
   // PART 15:   INCREMENT NEXT_STEP IF FALSE
   // ======================================================================================
   22: XIO(EdDSA_STATES[8].CMD.15)XIO(EdDSA_STATES[8].DONE.15)ADD(EdDSA_STATES[8].STEP,1,EdDSA_STATES[8].NEXT_STEP)OTL(EdDSA_STATES[8].DONE.15);
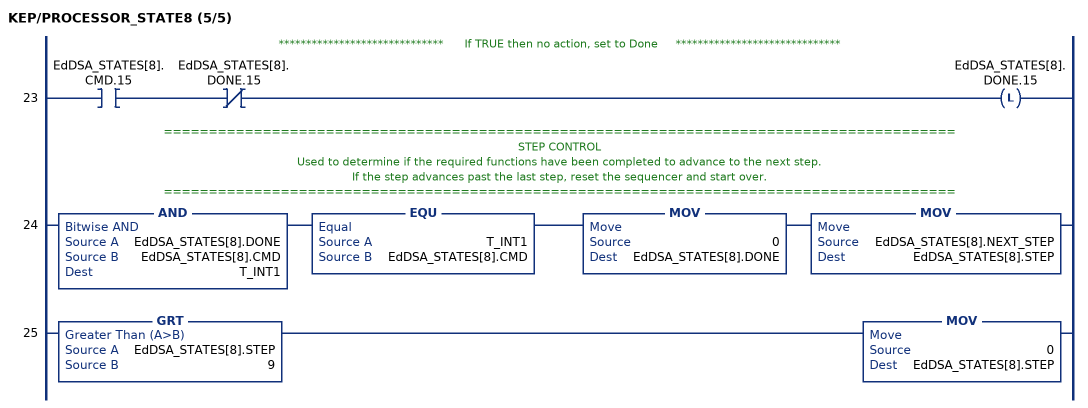
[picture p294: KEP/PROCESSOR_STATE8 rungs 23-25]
   // ******************************      If TRUE then no action, set to Done     ******************************
   23: XIC(EdDSA_STATES[8].CMD.15)XIO(EdDSA_STATES[8].DONE.15)OTL(EdDSA_STATES[8].DONE.15);
   // ========================================================================================
   // STEP CONTROL
   // Used to determine if the required functions have been completed to advance to the next step.
   // If the step advances past the last step, reset the sequencer and start over.
   // ========================================================================================
   24: AND(EdDSA_STATES[8].DONE,EdDSA_STATES[8].CMD,T_INT1)EQU(T_INT1,EdDSA_STATES[8].CMD)MOV(0,EdDSA_STATES[8].DONE)MOV(EdDSA_STATES[8].NEXT_STEP,EdDSA_STATES[8].STEP);
   25: GRT(EdDSA_STATES[8].STEP,9)MOV(0,EdDSA_STATES[8].STEP);
END_ROUTINE
